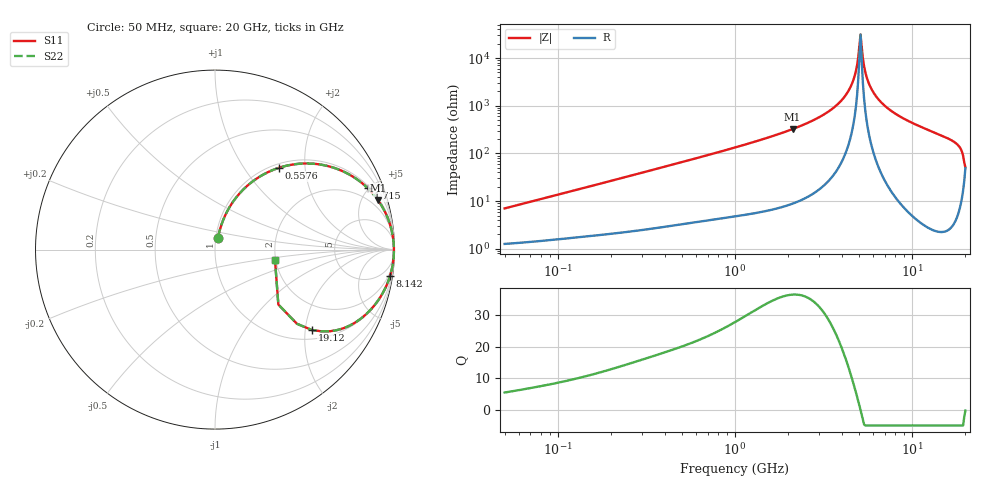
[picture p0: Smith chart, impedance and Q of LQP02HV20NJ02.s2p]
!Murata Part Number: LQP02HV20NJ02
!These Parameters are Measured in Series Mode Connection
!  o--[Z]--o
!Port1  Port2
!  o-------o
!Freq. Start=50[MHz] Stop=20[GHz], 401[Steps]
# Hz S RI R 50
!Freq.(Hz) S11(Real) S11(Imag) S21(Real) S21(Imag) S12(Real) S12(Imag) S22(Real) S22(Imag)
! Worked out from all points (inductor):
!   401 points, 50 MHz to 20 GHz, reference 50 ohm
!   read as one part in series: L = 21.9 nH near 51.52 MHz
!   highest Q = 36.6 at 2.115 GHz (marker M1), where L = 24.4 nH
!   self-resonance near 5.041 GHz
!   S11 on the Smith chart (normalised r, x): 50 MHz: 1.03, +0.14; 557.6 MHz: 1.07, +1.46; 1.715 GHz: 1.14, +4.92; 8.142 GHz: 1, -13; 19.12 GHz: 1.23, -2.17; 20 GHz: 1.98, -0.26
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5e7  0.0171 0.0672  0.9829 -0.0672  0.9829 -0.0672  0.0171 0.0672
1.364002e8  0.0484 0.1716  0.9516 -0.1716  0.9516 -0.1716  0.0484 0.1716
3.721004e8  0.2073 0.378  0.7927 -0.378  0.7927 -0.378  0.2073 0.378
5.575697e8  0.356 0.4557  0.644 -0.4557  0.644 -0.4557  0.356 0.4557
1e9  0.6355 0.4637  0.3645 -0.4637  0.3645 -0.4637  0.6355 0.4637
1.714689e9  0.8514 0.3418  0.1486 -0.3418  0.1486 -0.3418  0.8514 0.3418
2.114743e9  0.907 0.2771  0.093 -0.2771  0.093 -0.2771  0.907 0.2771
2.728004e9  0.9539 0.1958  0.0461 -0.1958  0.0461 -0.1958  0.9539 0.1958
3.572216e9  0.9832 0.1106  0.0168 -0.1106  0.0168 -0.1106  0.9832 0.1106
4.275624e9  0.9933 0.0549  0.00668 -0.0549  0.00668 -0.0549  0.9933 0.0549
4.677679e9  0.9959 0.0273  0.00413 -0.0273  0.00413 -0.0273  0.9959 0.0273
4.966507e9  0.9967 0.00888  0.00332 -0.00888  0.00332 -0.00888  0.9967 0.00888
5.117541e9  0.9968 -0.00033  0.00317 0.00033  0.00317 0.00033  0.9968 -0.00033
5.273168e9  0.9968 -0.00955  0.0032 0.00955  0.0032 0.00955  0.9968 -0.00955
5.515528e9  0.9964 -0.0234  0.00357 0.0234  0.00357 0.0234  0.9964 -0.0234
5.856089e9  0.9953 -0.042  0.00469 0.042  0.00469 0.042  0.9953 -0.042
7.442007e9  0.9833 -0.1175  0.0167 0.1175  0.0167 0.1175  0.9833 -0.1175
8.141811e9  0.9754 -0.1466  0.0246 0.1466  0.0246 0.1466  0.9754 -0.1466
1.573793e10  0.8148 -0.3829  0.1852 0.3829  0.1852 0.3829  0.8148 -0.3829
1.800918e10  0.6994 -0.4433  0.3006 0.4433  0.3006 0.4433  0.6994 -0.4433
1.912117e10  0.5398 -0.4479  0.4602 0.4479  0.4602 0.4479  0.5398 -0.4479
2e10  0.3343 -0.0584  0.6657 0.0584  0.6657 0.0584  0.3343 -0.0584
